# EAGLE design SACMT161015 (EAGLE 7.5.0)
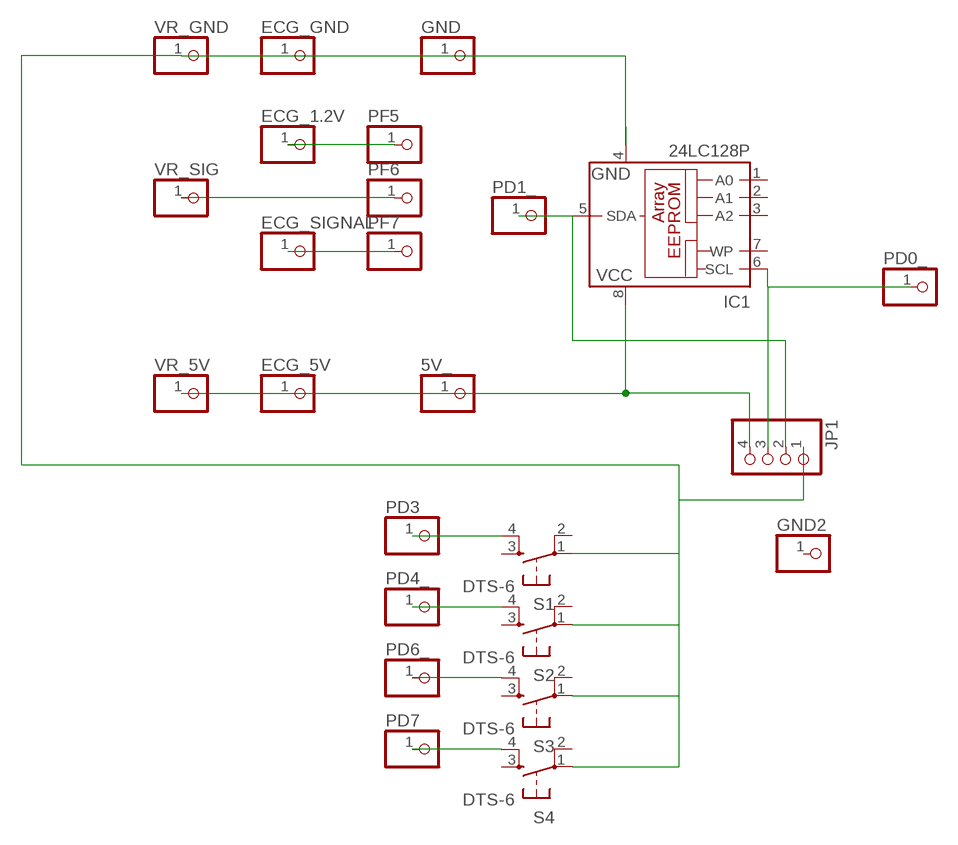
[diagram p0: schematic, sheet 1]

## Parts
5V_  PINHD-1X1  [1X01]
ECG_1.2V  PINHD-1X1  [1X01]
ECG_5V  PINHD-1X1  [1X01]
ECG_GND  PINHD-1X1  [1X01]
ECG_SIGNAL  PINHD-1X1  [1X01]
GND  PINHD-1X1  [1X01]
GND2  PINHD-1X1  [1X01]
IC1  24LC128P  [DIL8]
JP1  PINHD-1X4  [1X04]
PD0_  PINHD-1X1  [1X01]
PD1_  PINHD-1X1  [1X01]
PD3  PINHD-1X1  [1X01]
PD4_  PINHD-1X1  [1X01]
PD6_  PINHD-1X1  [1X01]
PD7  PINHD-1X1  [1X01]
PF5  PINHD-1X1  [1X01]
PF6  PINHD-1X1  [1X01]
PF7  PINHD-1X1  [1X01]
S1  DTS-6  [DTS-6]
S2  DTS-6  [DTS-6]
S3  DTS-6  [DTS-6]
S4  DTS-6  [DTS-6]
VR_5V  PINHD-1X1  [1X01]
VR_GND  PINHD-1X1  [1X01]
VR_SIG  PINHD-1X1  [1X01]

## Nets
N$1: IC1.5(SDA) JP1.2 PD1_.1
N$2: 5V_.1 ECG_5V.1 IC1.8(VCC) JP1.4 VR_5V.1
N$3: IC1.6(SCL) JP1.3 PD0_.1
N$4: ECG_GND.1 GND.1 IC1.4(GND) JP1.1 S1.1 S2.1 S3.1 S4.1 VR_GND.1
N$6: ECG_SIGNAL.1 PF7.1
N$7: ECG_1.2V.1 PF5.1
N$8: PF6.1 VR_SIG.1
N$9: PD3.1 S1.4
N$10: PD4_.1 S2.4
N$11: PD6_.1 S3.4
N$12: PD7.1 S4.4
Unconnected: GND2.1 IC1.1(A0) IC1.2(A1) IC1.3(A2) IC1.7(WP) S1.2 S1.3 S2.2 S2.3 S3.2 S3.3 S4.2 S4.3

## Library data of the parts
5V_ ECG_1.2V ECG_5V ECG_GND ECG_SIGNAL GND GND2 PD0_ PD1_ PD3 PD4_ PD6_ PD7 PF5-PF7 VR_5V VR_GND VR_SIG = pinhead:PINHD-1X1: PIN HEADER
IC1 = microchip:24*: Serial EEPROM I2C; MF: MICROCHIP; MPN: 24LC128-I/P; OC_FARNELL: 9757929; OC_NEWARK: 12C2007
JP1 = pinhead:PINHD-1X4: PIN HEADER
S1-S4 = switch-tact:DTS-6

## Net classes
0 default: width 0.406 mm

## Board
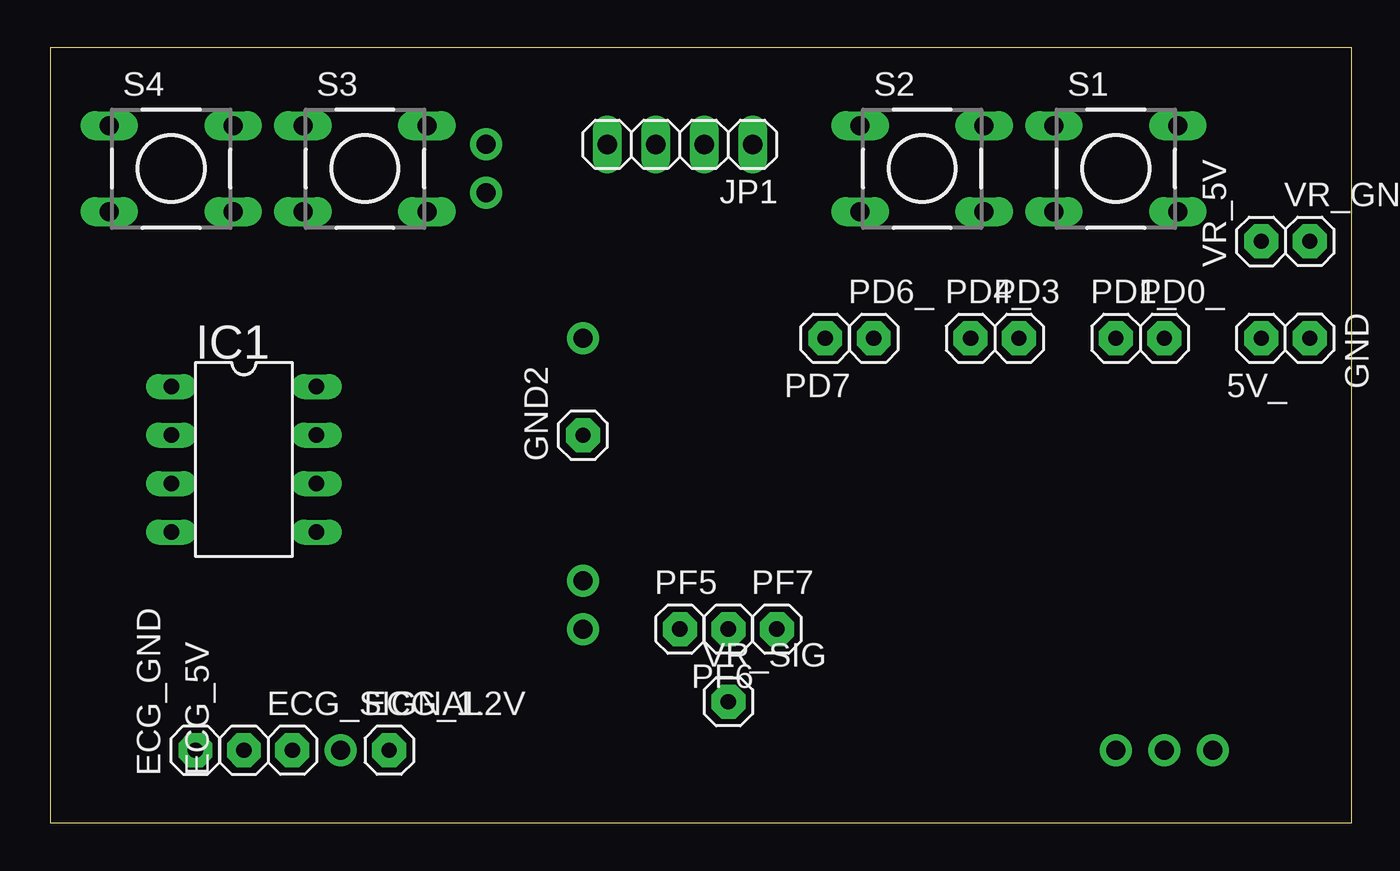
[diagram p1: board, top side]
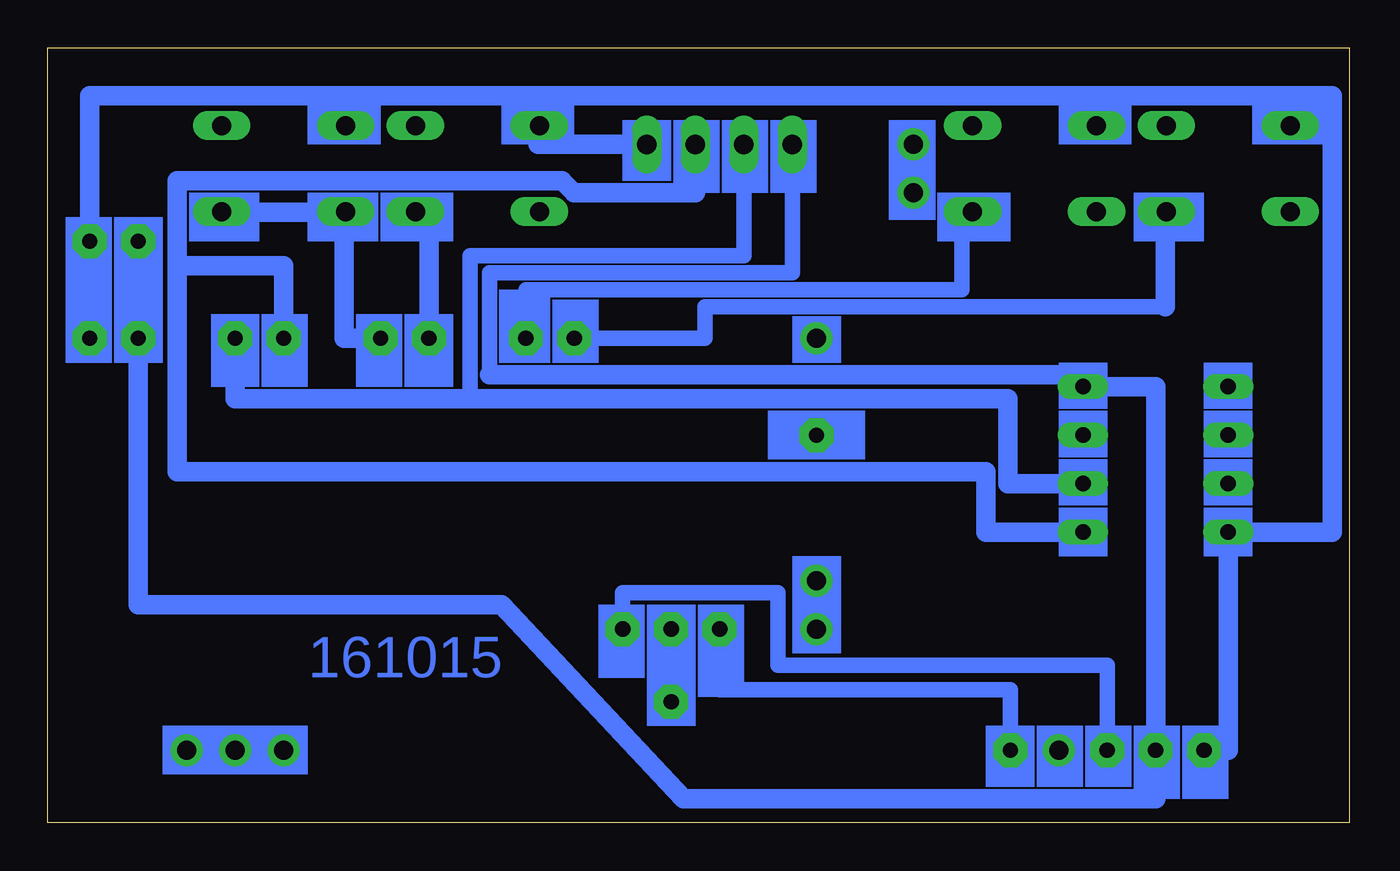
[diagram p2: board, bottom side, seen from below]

Size 68.25 x 40.63 mm. Coordinates in mm from the lower left corner, seen from the top.
Outline: 0,0 68.25,0 68.25,40.63 0,40.63 0,0
Copper layers (1*16): Top 0.035mm / dielectric 1.5mm / Bottom 0.035mm
Design rules "default *": minimum track width 20mil, minimum drill 24mil, track to track 8mil, track to pad 8mil, pad to pad 8mil, via to via 8mil, smd to smd 8mil, copper to edge 40mil, drill to drill 8mil, minimum pad ring 10mil, minimum via ring 8mil, stop-mask expansion 4mil, vias tented up to drill 0mil, thermal gap 10mil

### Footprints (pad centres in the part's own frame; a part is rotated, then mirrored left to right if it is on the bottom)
1X01 = drill 0.8 pad 1.778 octagon: 1 0,0
DIL8 = drill 0.813 long: 1 -3.81,-3.81; 2 -1.27,-3.81; 3 1.27,-3.81; 4 3.81,-3.81; 5 3.81,3.81; 6 1.27,3.81; 7 -1.27,3.81; 8 -3.81,3.81
1X04 = drill 1.016 long: 1 -3.81,0; 2 -1.27,0; 3 1.27,0; 4 3.81,0
DTS-6 = drill 1 long: 1 -3.25,2.25; 2 3.25,2.25; 3 -3.25,-2.25; 4 3.25,-2.25

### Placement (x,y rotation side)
5V_  63.5,25.4 180 top
ECG_1.2V  17.78,3.81 0 top
ECG_5V  10.16,3.81 90 top
ECG_GND  7.62,3.81 90 top
ECG_SIGNAL  12.7,3.81 0 top
GND  66.04,25.4 270 top
GND2  27.94,20.32 90 top
IC1  10.16,19.05 270 top
JP1  33.02,35.56 180 top
PD0_  58.42,25.4 0 top
PD1_  55.88,25.4 0 top
PD3  50.8,25.4 0 top
PD4_  48.26,25.4 0 top
PD6_  43.18,25.4 0 top
PD7  40.64,25.4 180 top
PF5  33.02,10.16 0 top
PF6  35.56,10.16 180 top
PF7  38.1,10.16 0 top
S1  55.88,34.29 0 top
S2  45.72,34.29 0 top
S3  16.51,34.29 0 top
S4  6.35,34.29 0 top
VR_5V  63.5,30.48 90 top
VR_GND  66.04,30.48 0 top
VR_SIG  35.56,6.35 0 top

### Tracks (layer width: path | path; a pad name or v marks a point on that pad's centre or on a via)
N$1
  Bottom 1.016: IC1.5 19.05,15.24 19.05,18.41 61.47,18.41 61.47,29.21 | 61.47,29.21 55.88,29.21 PD1_.1 | JP1.2 34.29,33.02 40.64,33.02 41.27,33.66 61.47,33.66 61.47,29.21
N$2
  Bottom 0.813: JP1.4 29.21,28.83 45.09,28.83 45.09,23.49
  Bottom 1.016: VR_5V.1 5V_.1 63.5,11.43 44.45,11.43 34.92,1.27 10.16,1.27 ECG_5V.1 10.16,22.86 IC1.8 14.61,23.49 45.09,23.49
N$3
  Bottom 0.813: JP1.3 31.75,29.72 46.1,29.72 46.1,22.23
  Bottom 1.016: IC1.6 17.91,17.78 17.91,22.23 46.1,22.23 58.42,22.23 PD0_.1
N$4
  Bottom 0.508: 3.17,38.1 3.17,36.83 S4.1 | 13.46,38.1 13.34,38.1 | 13.46,36.83 S3.1 13.34,36.83 | 42.55,35.56 42.55,36.2 | 52.7,36.83 S1.1
  Bottom 0.813: ECG_GND.1 6.35,3.81 | 42.55,36.2 S2.1 | 13.34,38.1 13.34,36.83
  Bottom 1.016: 6.35,3.81 IC1.4 0.89,15.24 0.89,38.1 3.05,38.1 S4.1 | 13.34,38.1 3.17,38.1 | 13.46,36.83 13.46,38.1 42.55,38.1 | GND.1 VR_GND.1 66.04,38.1 52.7,38.1 | JP1.1 42.55,35.56 | 52.7,38.1 52.7,36.83 | 42.55,38.1 52.7,38.1 | 42.55,38.1 42.55,36.83 S2.1
N$5  (via drill 1 pad 1.68)
  other vias: 22.86,35.56
N$6
  Bottom 0.813: ECG_SIGNAL.1 12.7,8.26 29.97,8.26 29.97,12.06 38.1,12.06 PF7.1
N$7
  Bottom 0.813: ECG_1.2V.1 17.78,6.98 33.02,6.98 PF5.1
N$8
  Bottom 0.813: VR_SIG.1 PF6.1
N$9
  Bottom 0.508: 59.05,32 S1.4
  Bottom 1.016: 59.05,32 52.7,32 52.7,25.4 PD3.1
N$10
  Bottom 0.813: 48.26,32 S2.4
  Bottom 1.016: PD4_.1 48.26,32
N$11
  Bottom 0.813: PD6_.1 43.18,27.94 20.32,27.94 20.32,31.75 S3.4
N$12
  Bottom 0.508: 9.65,31.75 S4.4
  Bottom 0.813: 9.65,27.05 33.78,27.05 33.78,25.4 PD7.1
  Bottom 1.016: 9.65,27.05 9.65,31.75
N$13  (via drill 1 pad 1.68)
  other vias: 22.86,33.02
N$14  (via drill 1 pad 1.68)
  other vias: 27.94,25.4
N$15  (via drill 1 pad 1.68)
  other vias: 27.94,12.7
N$16  (via drill 1 pad 1.68)
  other vias: 55.88,3.81
N$17  (via drill 1 pad 1.68)
  other vias: 58.42,3.81
N$18  (via drill 1 pad 1.68)
  other vias: 15.24,3.81
N$19  (via drill 1 pad 1.68)
  other vias: 60.96,3.81
N$20  (via drill 1 pad 1.68)
  other vias: 27.94,10.16
(copper drawn outside any net)
  shapes: Bottom area x42

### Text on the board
Bottom: 161015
